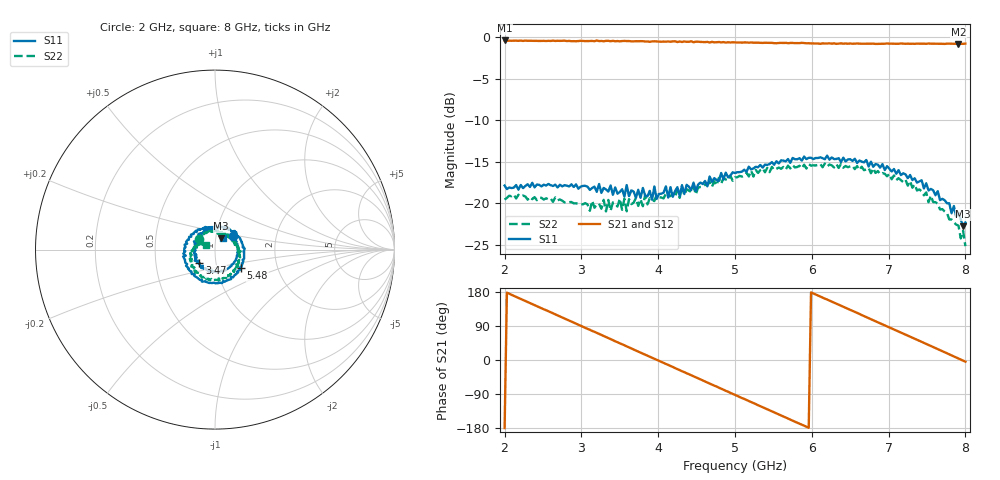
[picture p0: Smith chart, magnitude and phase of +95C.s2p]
!Agilent Technologies,E8361C,US49010292,A.09.42.06
!Agilent E8361C: A.09.42.06
!Date: Tuesday, January 14, 2025 01:51:27
!Correction: S11(Full 2 Port(1,2))
!S21(Full 2 Port(1,2))
!S12(Full 2 Port(1,2))
!S22(Full 2 Port(1,2))
!S2P File: Measurements: S11, S21, S12, S22:
# Hz S  dB  R 50
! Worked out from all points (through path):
!   201 points, 2 GHz to 8 GHz, reference 50 ohm
!   highest |S21| = -0.42 dB at 2 GHz (marker M1); lowest = -0.8 dB at 7.91 GHz (marker M2)
!   group delay of S21, straight-line fit = 252 ps
!   lowest |S11| = -22.8 dB at 7.97 GHz (marker M3), VSWR 1.16, Z = 53.1 + j6.83 ohm
!   |S11| at or under -10 dB: start of sweep to end of sweep
!   |S22| runs from -25.2 to -15.2 dB; largest |S21 - S12| = 0.011
!   S11 on the Smith chart (normalised r, x): 2 GHz: 1.21, +0.19; 3.47 GHz: 0.83, -0.13; 5.48 GHz: 1.31, -0.27; 8 GHz: 1.08, +0.14
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2e9  -17.87 37.5  -0.42 -179.6  -0.46 -179.6  -19.56 145.6
2.3e9  -17.71 1.3  -0.46 153.1  -0.47 153.1  -19.57 129.0
2.6e9  -17.83 -31.4  -0.48 125.9  -0.48 125.7  -19.42 107.7
3.02e9  -17.91 -80.0  -0.48 87.8  -0.50 87.7  -20.12 85.5
3.47e9  -18.85 -139.4  -0.49 47.0  -0.51 46.7  -20.39 67.8
3.77e9  -19.35 -177.7  -0.50 19.8  -0.56 19.7  -19.51 45.2
4.01e9  -18.88 151.7  -0.55 -2.2  -0.56 -2.2  -19.27 38.0
4.22e9  -18.53 122.8  -0.52 -21.3  -0.57 -21.3  -19.24 31.7
4.52e9  -17.75 80.4  -0.57 -48.5  -0.62 -48.5  -18.11 12.4
4.76e9  -17.21 48.6  -0.63 -70.0  -0.62 -70.4  -17.85 -2.4
5e9  -16.36 21.7  -0.65 -92.1  -0.66 -92.0  -16.88 -18.5
5.24e9  -15.81 -2.8  -0.69 -113.8  -0.67 -113.9  -16.80 -34.8
5.48e9  -15.05 -34.9  -0.71 -135.5  -0.72 -135.6  -15.62 -51.1
5.75e9  -14.55 -61.1  -0.72 -159.9  -0.78 -160.0  -15.40 -68.3
6.02e9  -14.69 -92.0  -0.78 175.7  -0.78 175.7  -15.44 -89.0
6.29e9  -14.68 -121.6  -0.77 151.4  -0.81 151.2  -15.69 -107.2
6.56e9  -14.65 -150.8  -0.80 126.9  -0.79 126.8  -15.89 -126.3
7.01e9  -15.84 160.1  -0.80 86.2  -0.86 86.2  -16.47 -159.6
7.43e9  -17.24 112.9  -0.80 47.9  -0.81 47.9  -18.55 173.1
7.91e9  -21.12 67.3  -0.84 4.0  -0.83 4.0  -22.69 147.1
7.97e9  -22.78 61.6  -0.83 -1.5  -0.83 -1.6  -23.30 148.1
8e9  -22.32 54.5  -0.79 -4.4  -0.84 -4.3  -25.16 149.5
